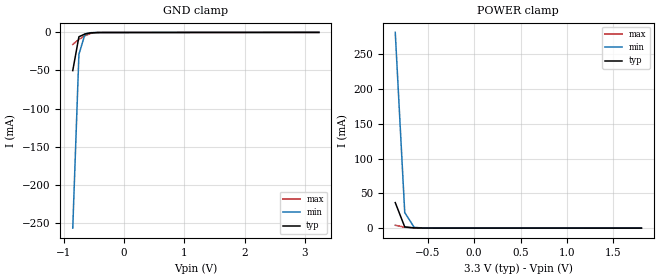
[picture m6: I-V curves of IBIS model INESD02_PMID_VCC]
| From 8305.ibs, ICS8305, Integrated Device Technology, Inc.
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[Model] INESD02_PMID_VCC
Model_type   Input
Polarity   Non-Inverting
Vinl = 0.8V
Vinh = 2.0V
|   typ   min   max
C_comp   2pF   1.5pF   2.5pF
|   typ   min   max
[Voltage range]   3.3V   3.135V   3.465V
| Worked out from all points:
|   GND clamp passes 1 mA (typ) near -0.58 V on its own axis
|   POWER clamp passes 1 mA (typ) near -0.69 V on its own axis
[GND_clamp]
|Voltage   I (typ)   I (min)   I (max)
|Note, modeling breaks down at 250mA and above.  This is well beyond the functional   |
|operating range of the device.  Should this scenario occur, catastrophic failure and   |
|possible damage to the device and/or board is of higher concern than the I-V curve   |
|behavior.  The IBIS checker will flag currents in excess of 10A with warnings.  Lines   |
|with currents in excess of 0.35 A have been commented out.  The points still remain|
|available to the user if the user desires to use them.   |
|-3.19794e+00   -7.34136e+00   -6.33783e+00   -9.01402e+00
|-3.09588e+00   -7.02359e+00   -6.07292e+00   -8.60887e+00
|-2.99381e+00   -6.70583e+00   -5.80804e+00   -8.20370e+00
|-2.89175e+00   -6.38807e+00   -5.54317e+00   -7.79853e+00
|-2.78969e+00   -6.07031e+00   -5.27833e+00   -7.39334e+00
|-2.68763e+00   -5.75255e+00   -5.01351e+00   -6.98814e+00
|-2.58557e+00   -5.43479e+00   -4.74871e+00   -6.58291e+00
|-2.48351e+00   -5.11702e+00   -4.48393e+00   -6.17766e+00
|-2.38144e+00   -4.79925e+00   -4.21917e+00   -5.77239e+00
|-2.27938e+00   -4.48147e+00   -3.95444e+00   -5.36709e+00
|-2.17732e+00   -4.16369e+00   -3.68974e+00   -4.96176e+00
|-2.07526e+00   -3.84591e+00   -3.42507e+00   -4.55640e+00
|-1.97320e+00   -3.52813e+00   -3.16044e+00   -4.15101e+00
|-1.87113e+00   -3.21035e+00   -2.89585e+00   -3.74559e+00
|-1.76907e+00   -2.89259e+00   -2.63132e+00   -3.34013e+00
|-1.66701e+00   -2.57484e+00   -2.36686e+00   -2.93464e+00
|-1.56495e+00   -2.25713e+00   -2.10248e+00   -2.52913e+00
|-1.46289e+00   -1.93946e+00   -1.83821e+00   -2.12360e+00
|-1.36082e+00   -1.62186e+00   -1.57408e+00   -1.71805e+00
|-1.25876e+00   -1.30437e+00   -1.31011e+00   -1.31251e+00
|-1.15670e+00   -9.87034e-01   -1.04636e+00   -9.07000e-01
|-1.05464e+00   -6.69908e-01   -7.82881e-01   -5.01565e-01
|-9.52577e-01   -3.53090e-01   -5.19770e-01   -9.63696e-02
-850.5mV  -50.08mA   -257.1mA   -15.69mA
-748.5mV  -5.694mA   -28.81mA   -9.243mA
-646.4mV  -1.98mA    -1.883mA   -4.221mA
-544.3mV  -498.6uA   -303.9uA   -1.102mA
-442.3mV  -134.6uA   -126.4uA   -188.1uA
3.232V    66.31uA    87.24uA    53.58uA
[Power_clamp]
|Voltage   I (typ)   I (min)   I (max)
|Note, modeling breaks down at 250mA and above.  This is well beyond the functional   |
|operating range of the device.  Should this scenario occur, catastrophic failure and   |
|possible damage to the device and/or board is of higher concern than the I-V curve   |
|behavior.  The IBIS checker will flag currents in excess of 10A with warnings.  Lines   |
|with currents in excess of 0.35 A have been commented out.  The points still remain|
|available to the user if the user desires to use them.   |
|-3.19794e+00   9.37738e+00   8.08501e+00   1.15363e+01
|-3.09588e+00   8.96843e+00   7.74460e+00   1.10142e+01
|-2.99381e+00   8.55949e+00   7.40424e+00   1.04921e+01
|-2.89175e+00   8.15058e+00   7.06394e+00   9.97001e+00
|-2.78969e+00   7.74169e+00   6.72370e+00   9.44786e+00
|-2.68763e+00   7.33283e+00   6.38353e+00   8.92569e+00
|-2.58557e+00   6.92400e+00   6.04342e+00   8.40351e+00
|-2.48351e+00   6.51521e+00   5.70338e+00   7.88131e+00
|-2.38144e+00   6.10646e+00   5.36342e+00   7.35911e+00
|-2.27938e+00   5.69777e+00   5.02353e+00   6.83691e+00
|-2.17732e+00   5.28913e+00   4.68374e+00   6.31471e+00
|-2.07526e+00   4.88057e+00   4.34405e+00   5.79253e+00
|-1.97320e+00   4.47209e+00   4.00446e+00   5.27039e+00
|-1.87113e+00   4.06372e+00   3.66499e+00   4.74829e+00
|-1.76907e+00   3.65547e+00   3.32566e+00   4.22626e+00
|-1.66701e+00   3.24736e+00   2.98648e+00   3.70432e+00
|-1.56495e+00   2.83943e+00   2.64747e+00   3.18251e+00
|-1.46289e+00   2.43171e+00   2.30865e+00   2.66088e+00
|-1.36082e+00   2.02424e+00   1.97005e+00   2.13948e+00
|-1.25876e+00   1.61708e+00   1.63171e+00   1.61839e+00
|-1.15670e+00   1.21029e+00   1.29365e+00   1.09770e+00
|-1.05464e+00   8.03937e-01   9.55928e-01   5.77542e-01
|-9.52577e-01   3.98139e-01   6.18603e-01   6.89658e-02
-850.5mV  36.74mA    281.8mA    4.124mA
-748.5mV  1.769mA    22.45mA    1.23mA
-646.4mV  325.6uA    1.081mA    262.5uA
-442.3mV  89.96uA    109.5uA    78.52uA
1.803V    -6.417uA   -12.35uA   -2.522uA
